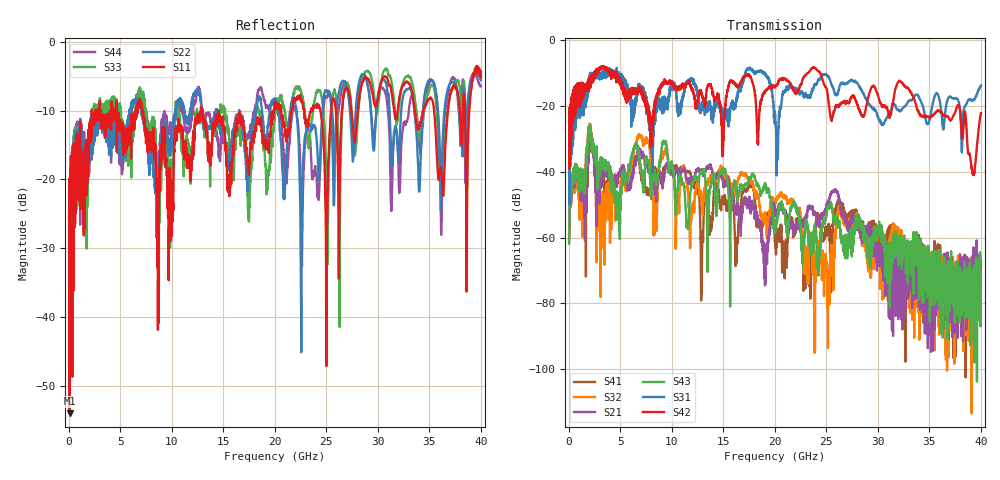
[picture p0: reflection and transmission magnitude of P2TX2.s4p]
!Agilent Technologies,N5245A,MY49151084,A.09.20.08
!Agilent N5245A: A.09.20.08
!Date: Thursday, March 01, 2012 14:44:25
!Correction: S11(Full 4 Port(1,2,3,4))
!S12(Full 4 Port(1,2,3,4))
!S13(Full 4 Port(1,2,3,4))
!S14(Full 4 Port(1,2,3,4))
!S21(Full 4 Port(1,2,3,4))
!S22(Full 4 Port(1,2,3,4))
!S23(Full 4 Port(1,2,3,4))
!S24(Full 4 Port(1,2,3,4))
!S31(Full 4 Port(1,2,3,4))
!S32(Full 4 Port(1,2,3,4))
!S33(Full 4 Port(1,2,3,4))
!S34(Full 4 Port(1,2,3,4))
!S41(Full 4 Port(1,2,3,4))
!S42(Full 4 Port(1,2,3,4))
!S43(Full 4 Port(1,2,3,4))
!S44(Full 4 Port(1,2,3,4))
!S4P File: Measurements: <S11,S12,S13,S14>,
!<S21,S22,S23,S24>,
!<S31,S32,S33,S34>,
!<S41,S42,S43,S44>:
# Hz S  dB  R 50
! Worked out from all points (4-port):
!   3996 points, 50 MHz to 40 GHz, reference 50 ohm
!   strongest paths, dB at 50 MHz, 10.04 GHz, 20.03 GHz, 30.02 GHz, 40 GHz:
!     S42: -25.0, -12.9, -14.3, -16.9, -22.3
!     S31: -24.7, -13.9, -22.7, -23.2, -13.9
!     S43: -61.9, -38.8, -56.9, -57.3, -71.4
!     S21: -59.2, -39.5, -51.2, -62.9, -75.8
!     S32: -55.9, -38.1, -49.8, -66.2, -66.8
!     S41: -61.2, -38.8, -60.0, -60.4, -74.1
!   lowest |S11| = -54.0 dB at 90 MHz (marker M1), VSWR 1.00, Z = 49.8 + j0.109 ohm
!   |S11| at or under -10 dB: start of sweep to 2.24 GHz; 7.192 GHz to 12.82 GHz (5.626 GHz wide, 56.2 % of centre); 14.56 GHz to 19.9 GHz (5.343 GHz wide, 31 % of centre)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
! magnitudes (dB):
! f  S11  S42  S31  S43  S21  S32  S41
! 50 MHz  -22.1  -25.0  -24.7  -61.9  -59.2  -55.9  -61.2
! 90 MHz  -54.0  -33.5  -50.0  -51.8  -51.9  -52.1  -52.8
! 2.04 GHz  -13.6  -14.6  -12.4  -26.7  -28.3  -26.0  -29.9
! 3.3 GHz  -11.8  -8.2  -11.0  -38.2  -40.7  -49.1  -41.8
! 6.93 GHz  -8.6  -14.5  -14.2  -37.8  -33.9  -29.2  -38.9
! 8.4 GHz  -14.8  -19.8  -24.6  -41.6  -45.4  -52.5  -38.8
! 40 GHz  -5.2  -22.3  -13.9  -71.4  -75.8  -66.8  -74.1
